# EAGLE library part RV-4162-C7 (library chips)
This ultra small RTC Module has been specially designed for miniature and cost sensitive high volume applications.
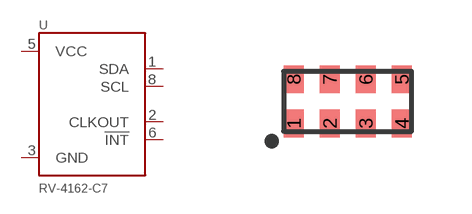
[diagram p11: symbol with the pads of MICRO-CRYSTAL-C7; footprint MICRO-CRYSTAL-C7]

Designator prefix U

## RV-4162-C7 (NEWARK: 09X0517)  [MICRO-CRYSTAL-C7]
1  SDA
2  CLKOUT
3  GND
5  VCC
6  !INT
8  SCL

## Footprint MICRO-CRYSTAL-C7 (pad centres in mm)
smd 0.5 x 0.7: 1 -1.35,-0.55; 2 -0.45,-0.55; 3 0.45,-0.55; 4 1.35,-0.55; 5 1.35,0.55; 6 0.45,0.55; 7 -0.45,0.55; 8 -1.35,0.55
